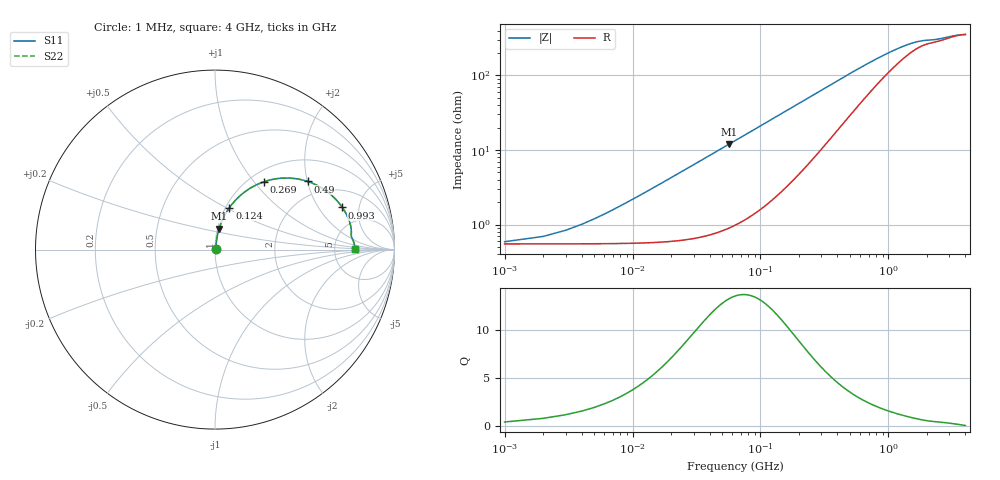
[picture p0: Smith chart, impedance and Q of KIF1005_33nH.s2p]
!version-2
!date-12.2020
!Series
# MHz S RI R 50
!Freq ReS11 ImS11 ReS21 ImS21 ReS12 ImS12 ReS22 ImS22
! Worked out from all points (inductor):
!   4000 points, 1 MHz to 4 GHz, reference 50 ohm
!   read as one part in series: L = 33.5 nH near 21 MHz
!   highest Q = 13.3 at 57 MHz (marker M1), where L = 33.4 nH
!   S11 on the Smith chart (normalised r, x): 1 MHz: 1.01, +0.00; 124 MHz: 1.04, +0.52; 269 MHz: 1.17, +1.13; 490 MHz: 1.56, +2.01; 993 MHz: 3.16, +3.36; 4 GHz: 8.10, +0.14
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1  0.00547 0.00208  0.9945 -0.00208  0.9945 -0.00208  0.00547 0.00208
11  0.00612 0.0229  0.9939 -0.0229  0.9939 -0.0229  0.00612 0.0229
24  0.00859 0.0498  0.9914 -0.0498  0.9914 -0.0498  0.00859 0.0498
29  0.01 0.06  0.99 -0.06  0.99 -0.06  0.01 0.06
41  0.0145 0.0843  0.9855 -0.0843  0.9855 -0.0843  0.0145 0.0843
57  0.0227 0.116  0.9773 -0.116  0.9773 -0.116  0.0227 0.116
86  0.0435 0.1705  0.9565 -0.1705  0.9565 -0.1705  0.0435 0.1705
124  0.0807 0.2343  0.9193 -0.2343  0.9193 -0.2343  0.0807 0.2343
154  0.1163 0.2774  0.8837 -0.2774  0.8837 -0.2774  0.1163 0.2774
188  0.1609 0.3177  0.8391 -0.3177  0.8391 -0.3177  0.1609 0.3177
269  0.2736 0.3784  0.7264 -0.3784  0.7264 -0.3784  0.2736 0.3784
366  0.3967 0.3989  0.6033 -0.3989  0.6033 -0.3989  0.3967 0.3989
490  0.5157 0.3799  0.4843 -0.3799  0.4843 -0.3799  0.5157 0.3799
668  0.6211 0.3257  0.3789 -0.3257  0.3789 -0.3257  0.6211 0.3257
815  0.6718 0.2811  0.3282 -0.2811  0.3282 -0.2811  0.6718 0.2811
993  0.7093 0.2349  0.2907 -0.2349  0.2907 -0.2349  0.7093 0.2349
1334  0.745 0.1681  0.255 -0.1681  0.255 -0.1681  0.745 0.1681
1657  0.7576 0.1232  0.2424 -0.1232  0.2424 -0.1232  0.7576 0.1232
2001  0.7595 0.0907  0.2405 -0.0907  0.2405 -0.0907  0.7595 0.0907
2667  0.7654 0.0601  0.2346 -0.0601  0.2346 -0.0601  0.7654 0.0601
3334  0.7761 0.0305  0.2239 -0.0305  0.2239 -0.0305  0.7761 0.0305
4000  0.7803 0.00348  0.2197 -0.00348  0.2197 -0.00348  0.7803 0.00348
